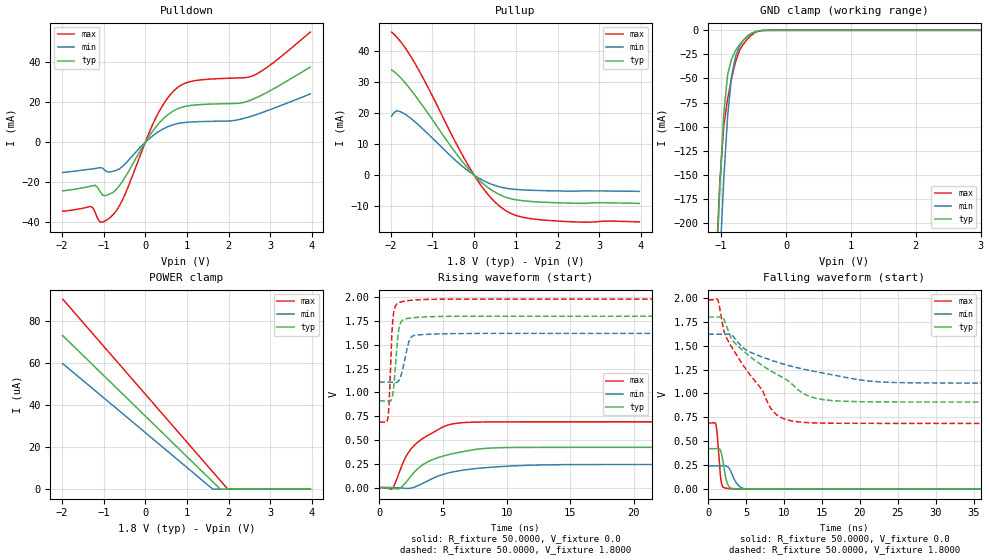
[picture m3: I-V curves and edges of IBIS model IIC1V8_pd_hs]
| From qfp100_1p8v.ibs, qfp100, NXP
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[Model] IIC1V8_pd_hs
|   Model IIC1V8_pd_hs
| This model was characterised for following simulation conditions:
| External (pad) voltage:
|   - Typ: 1.8V,   - Min: 1.62V,   - Max: 1.98V
| Library cells for typ/min/max conditions are connected as defined below:
|  IO - External Pad
|  A - Core Input
|  EN - Output Buffer Enable
|  BOOST - vdde
|  EGP - vdd
|  EHS - vdd
|  ENZI - vdd
|  EPD - vdd
|  EPUN - vdd
|  ZI - NC
|  ZIF - NC
|  gnd - gnd
|  gnde - gnde
|  vdd - vdd
|  vdde - vdde
| All other pins connected to ground
Model_type I/O
Polarity   Non-Inverting
Enable   Active-Low
Vinl =   0.5400V
Vinh =   1.2600V
Vmeas =  0.9000V
Cref =   0.0F
Rref =   1.0000k
Vref =   0.0V
C_comp   3.6136pF   3.4665pF   3.7543pF
|C_comp_pullup   0.9376pF   0.9158pF   0.9440pF
|C_comp_pulldown   2.3253pF   2.4782pF   2.1796pF
[Model Spec]
| variable   typ   min   max
Vinh   0.5400V   0.4860V   0.5940V
Vinl   1.2600V   1.1340V   1.3860V
Vmeas   0.9000V   0.8100V   0.9900V
[Temperature Range]   25.0000   0.1250k   -40.0000
[Voltage Range]   1.8000V   1.6200V   1.9800V
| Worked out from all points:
|   slope of the pulldown table from 0 to 0.27 V, typ, clamps not added: 33.4 ohm
|   slope of the pullup table from 0 to 0.27 V, typ, clamps not added: 80.7 ohm
|   GND clamp passes 1 mA (typ) near -0.44 V on its own axis
|   rising waveform, R_fixture 50.0000, V_fixture 0.0: 20-80 % time 2.94ns typ, 3.7ns min, 2.37ns max; typ from 0 V to 0.423 V
|   rising waveform, R_fixture 50.0000, V_fixture 1.8000: 20-80 % time 334ps typ, 515ps min, 244ps max; typ from 0.91 V to 1.8 V
|   falling waveform, R_fixture 50.0000, V_fixture 0.0: 20-80 % time 582ps typ, 939ps min, 399ps max; typ from 0.423 V to 0 V
|   falling waveform, R_fixture 50.0000, V_fixture 1.8000: 20-80 % time 8.41ns typ, 11.2ns min, 5.74ns max; typ from 1.8 V to 0.91 V
[Pulldown]
|Voltage   I(typ)   I(min)   I(max)
-1.98V    -24.22mA   -15.04mA   -34.42mA
-1.32V    -21.94mA   -13.41mA   -32.06mA
-1.2V     -21.45mA   -13.05mA   -35.06mA
-1.08V    -24.63mA   -12.6mA    -39.9mA
-900mV    -26.23mA   -14.78mA   -38.53mA
-720mV    -24.07mA   -14.13mA   -34.99mA
-540mV    -19.33mA   -11.9mA    -28.53mA
300mV     8.856mA    5.096mA    14.12mA
720mV     16.26mA    9.117mA    26.48mA
1.14V     18.6mA     10.26mA    30.69mA
2.58V     21.55mA    13.34mA    33.32mA
3.96V     37.7mA     24.26mA    55.17mA
[Pullup]
|Voltage   I(typ)   I(min)   I(max)
-1.98V    33.82mA    18.95mA    45.98mA
-1.86V    32.54mA    20.66mA    44.41mA
-1.62V    29.1mA     19.25mA    40.23mA
-1.2V     21.63mA    14.45mA    30.58mA
-420mV    6.731mA    4.413mA    9.887mA
0V        -16.46nA   -7.885nA   -32.77nA
360mV     -4.265mA   -2.608mA   -6.666mA
660mV     -6.57mA    -3.917mA   -10.5mA
1.02V     -7.945mA   -4.606mA   -13.01mA
1.56V     -8.618mA   -4.934mA   -14.29mA
2.64V     -9.058mA   -5.064mA   -15.11mA
3.96V     -9.081mA   -5.209mA   -15.04mA
[GND_clamp]
|Voltage   I(typ)   I(min)   I(max)
-1.98V    -2.104A    -2.075A    -2.136A
-1.08V    -259.3mA   -333mA     -246.9mA
-1.02V    -161.8mA   -238.7mA   -157.1mA
-960mV    -86.75mA   -154.7mA   -99.47mA
-900mV    -45.96mA   -88.82mA   -71.06mA
-840mV    -29.91mA   -48mA      -50.26mA
-780mV    -21.16mA   -27.65mA   -32.99mA
-720mV    -15.17mA   -16.88mA   -21.27mA
-660mV    -10.57mA   -10.24mA   -14.57mA
-540mV    -3.796mA   -3.405mA   -5.301mA
-300mV    -21.69uA   -40.85uA   -23.15uA
3.96V     0A         0A         0A
[POWER_clamp]
|Voltage   I(typ)   I(min)   I(max)
-1.98V    73.06uA    59.72uA    90.42uA
1.62V     3.484uA    0A         8.225uA
1.8V      0A         0A         4.113uA
1.98V     0A         0A         0A
3.96V     0A         0A         0A
[Ramp]
| variable   typ   min   max
dV/dt_r  0.2537/2.9388n   0.1456/3.6995n   0.4146/2.3712n
dV/dt_f  0.5332/8.4066n   0.3066/11.2331n   0.7749/5.7392n
R_load = 50.0000
[Rising Waveform]
R_fixture= 50.0000
V_fixture= 0.0
V_fixture_min= 0.0
V_fixture_max= 0.0
|time   V(typ)   V(min)   V(max)
0s        583.8pV    50.78nV    39.11pV
1.054ns   -4.514mV   242.5uV    -9.548mV
1.61ns    -8.523mV   -2.31mV    174.3mV
2.273ns   83.48mV    -8.964mV   364.5mV
2.96ns    191.1mV    15.43mV    468.9mV
3.647ns   258.5mV    59.9mV     534.9mV
5.688ns   353.4mV    162.2mV    666.4mV
8.866ns   415.9mV    214.9mV    689.9mV
20.33ns   422.8mV    242.4mV    690.9mV
1us       422.9mV    242.6mV    691mV
[Rising Waveform]
R_fixture= 50.0000
V_fixture= 1.8000
V_fixture_min= 1.6200
V_fixture_max= 1.9800
|time   V(typ)   V(min)   V(max)
0s        910.3mV    1.108V     687.5mV
691.8ps   908.2mV    1.108V     744.4mV
790.1ps   905.2mV    1.109V     926.9mV
1.021ns   951.9mV    1.107V     1.683V
1.287ns   1.301V     1.102V     1.909V
1.516ns   1.645V     1.119V     1.94V
1.779ns   1.751V     1.209V     1.952V
2.54ns    1.781V     1.583V     1.967V
4.645ns   1.796V     1.613V     1.977V
1us       1.799V     1.619V     1.979V
[Falling Waveform]
R_fixture= 50.0000
V_fixture= 0.0
V_fixture_min= 0.0
V_fixture_max= 0.0
|time   V(typ)   V(min)   V(max)
0s        422.9mV    242.6mV    691mV
1.028ns   422.9mV    242.6mV    672mV
1.233ns   425.5mV    242.6mV    535.2mV
1.608ns   406.8mV    242.6mV    141.8mV
1.876ns   324.7mV    244.1mV    31.7mV
2.285ns   129.3mV    244.3mV    11.56mV
2.692ns   32.3mV     224.7mV    6.307mV
3.63ns    4.191mV    74.61mV    1.844mV
4.418ns   1.837mV    14.45mV    786.2uV
1us       17.18nV    79.91nV    9.929nV
[Falling Waveform]
R_fixture= 50.0000
V_fixture= 1.8000
V_fixture_min= 1.6200
V_fixture_max= 1.9800
|time   V(typ)   V(min)   V(max)
0s        1.799V     1.619V     1.979V
1.244ns   1.799V     1.619V     1.982V
1.89ns    1.801V     1.619V     1.717V
2.453ns   1.696V     1.621V     1.575V
3.833ns   1.502V     1.542V     1.391V
8.766ns   1.214V     1.335V     796.1mV
12.87ns   986.9mV    1.25V      696.5mV
15.31ns   934.7mV    1.211V     690mV
35.03ns   910.7mV    1.109V     687.6mV
1us       910.3mV    1.108V     687.5mV
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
